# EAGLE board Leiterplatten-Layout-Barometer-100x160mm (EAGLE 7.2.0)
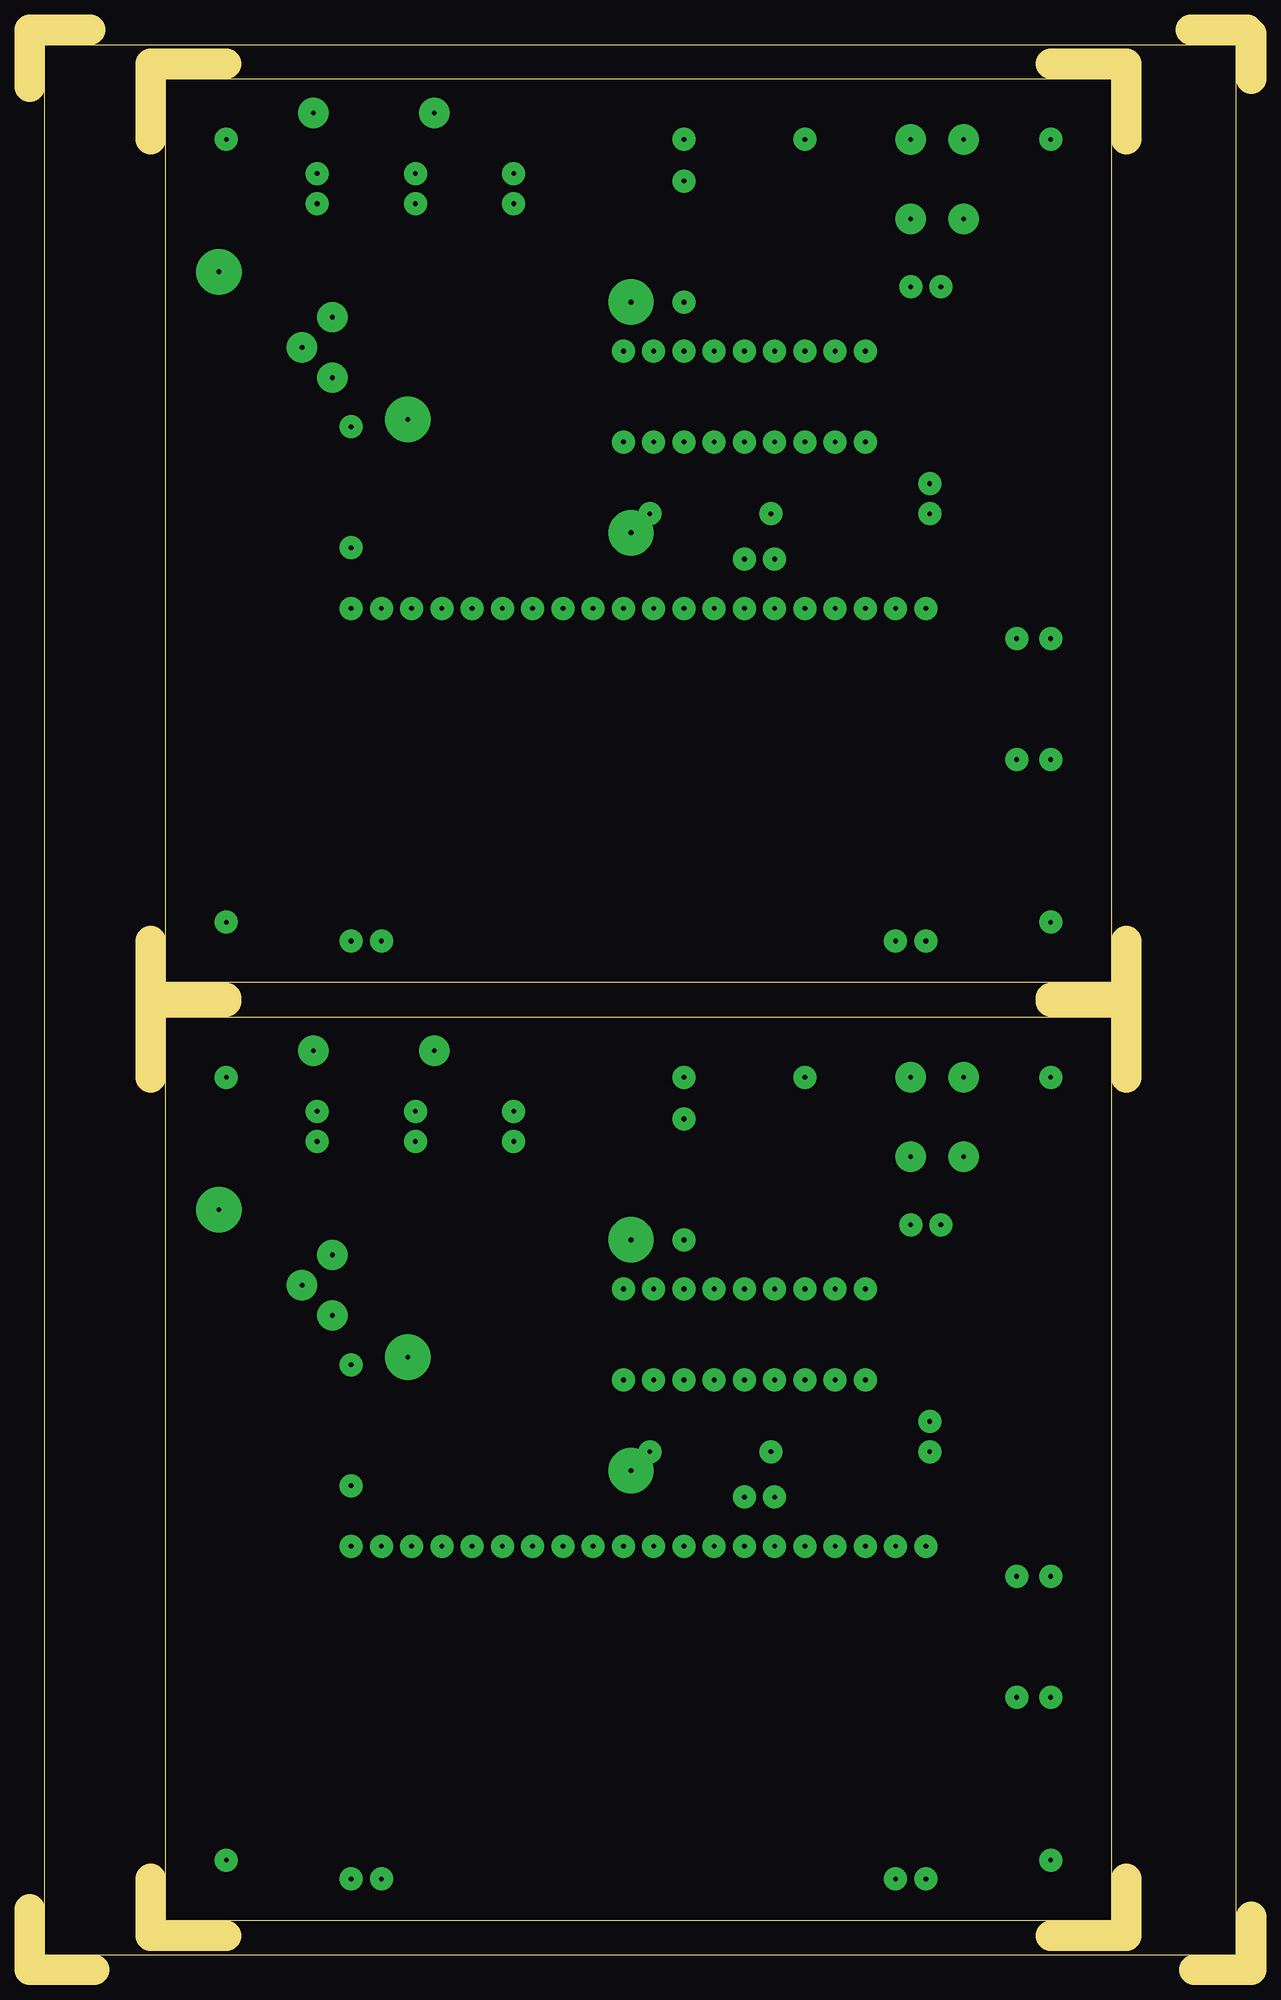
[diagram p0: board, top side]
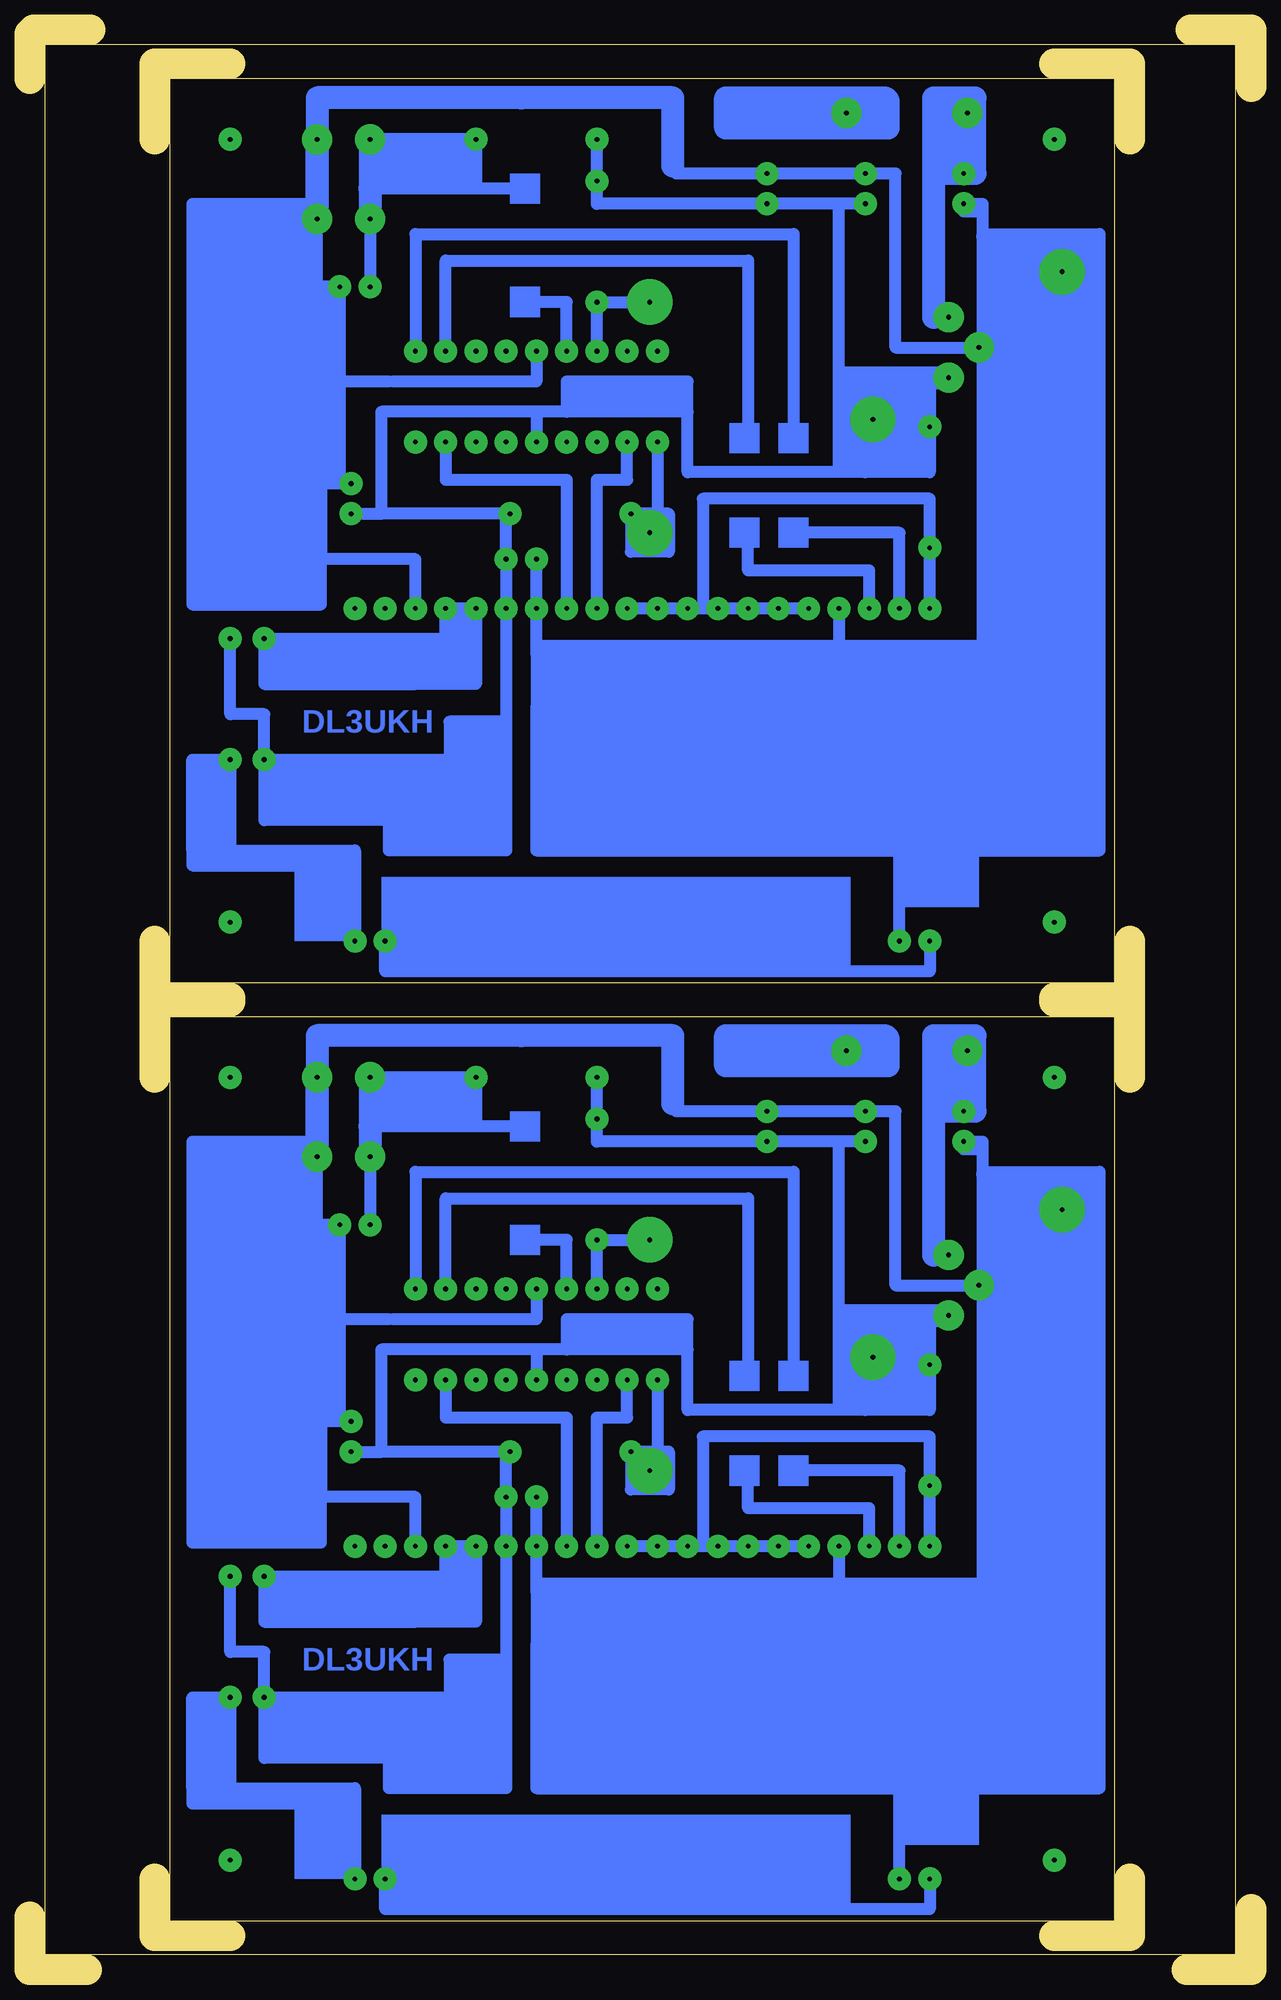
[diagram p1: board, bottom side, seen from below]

Size 102.55 x 162.88 mm. Coordinates in mm from the lower left corner, seen from the top.
Outline: 5.4,0 0.32,0
Outline: 0,0 0,5.08
Outline: 97.79,0 102.55,0 102.55,4.45
Outline: 5.08,162.88 0,162.88 0,158.12
Outline: 102.55,158.75 102.55,162.56
Outline: 97.47,162.88 102.23,162.88
Outline: 92.08,153.67 92.08,160.02 85.72,160.02
Outline: 92.08,86.36 92.08,81.6 85.72,81.6
Outline: 16.51,81.6 10.16,81.6 10.16,86.36
Outline: 10.16,153.67 10.16,160.02 16.51,160.02
Outline: 92.08,74.93 92.08,81.28 85.72,81.28
Outline: 92.08,7.62 92.08,2.86 85.72,2.86
Outline: 16.51,2.86 10.16,2.86 10.16,7.62
Outline: 10.16,74.93 10.16,81.28 16.51,81.28
Outline: 1.27,1.27 101.28,1.27 101.28,161.61 1.27,161.61 1.27,1.27
Outline: 90.8,158.75 90.8,82.87 11.43,82.87 11.43,158.75 90.8,158.75
Outline: 90.8,80.01 90.8,4.13 11.43,4.13 11.43,80.01 90.8,80.01
Copper layers (1*16): Top 0.035mm / dielectric 1.5mm / Bottom 0.035mm
Design rules "default": minimum track width 10mil, minimum drill 24mil, track to track 8mil, track to pad 8mil, pad to pad 8mil, via to via 8mil, smd to smd 8mil, copper to edge 40mil, drill to drill 8mil, minimum pad ring 10mil, minimum via ring 8mil, stop-mask expansion 4mil, vias tented up to drill 0mil, thermal gap 10mil

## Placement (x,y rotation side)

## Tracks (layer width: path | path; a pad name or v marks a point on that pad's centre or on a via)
S$1  (via drill 0.4 pad 1.93)
  Bottom 1.016: v26.99,7.62 26.99,5.08 72.71,5.08 v72.71,7.62
S$2  (via drill 0.4 pad 1.93)
  other vias: 42.23,114.3
S$3  (via drill 0.4 pad 1.93)
  Bottom 1.016: v26.99,86.36 26.99,83.82 72.71,83.82 v72.71,86.36
S$4  (via drill 0.4 pad 1.93, 0.4 pad 2.54)
  Bottom 1.016: 21.91,136.21 v22.86,136.21 29.84,136.21 29.84,150.81 v32.38,150.81 48.26,150.81 | 21.91,136.21 21.91,108.9 23.5,96.52 | v29.53,86.36 29.53,96.52 | 29.53,96.52 60.01,96.52 | 60.01,96.52 60.01,106.05 | 60.01,110.49 60.01,111.12 | 60.01,111.12 v60.01,114.3 v60.01,118.43 | 60.01,96.52 60.01,93.98 23.81,93.98 | 23.5,96.52 29.53,96.52 | 23.5,96.52 23.5,93.98 12.7,93.98 12.7,145.73 22.54,145.73 | 51.75,110.49 50.8,110.49 50.8,106.05 60.01,106.05 | 51.75,110.49 60.01,110.49 | 60.01,110.49 60.01,106.05 | 51.75,109.22 51.75,110.49 | v15.88,142.56 22.54,145.73 | 21.91,136.21 22.54,145.73 | 22.22,111.12 60.01,111.12
S$5
  Bottom 1.016: 34.61,114.3 34.61,95.57
S$6  (via drill 0.4 pad 1.93, 0.4 pad 3.81)
  Bottom 1.016: v54.93,135.89 v54.93,140.02 v50.48,140.02
S$7  (via drill 0.4 pad 1.93)
  other vias: 42.23,35.56
S$8  (via drill 0.4 pad 1.93)
  other vias: 16.51,87.95
S$9  (via drill 0.4 pad 1.93)
  other vias: 16.51,153.67
S$10
  Bottom 1.016: 75.56,156.84 75.56,157.48 | 75.56,157.48 78.74,157.48 | 61.28,157.16 58.42,157.48 | 58.42,157.48 75.56,157.48 | 58.42,157.48 48.58,157.48 48.58,157.16
  Bottom 1.93: 61.28,157.16 78.1,157.16 | 48.58,151.45 48.58,157.16 78.42,157.16 78.42,147
S$11  (via drill 0.4 pad 1.93)
  other vias: 44.77,114.3
S$12  (via drill 0.4 pad 1.93)
  other vias: 57.47,128.27
S$13  (via drill 0.4 pad 1.93)
  other vias: 44.77,35.56
S$14  (via drill 0.4 pad 1.93)
  Bottom 1.016: v54.93,114.3 54.93,125.09 52.39,125.09 v52.39,128.27
S$15  (via drill 0.4 pad 1.93)
  other vias: 34.61,114.3
S$16  (via drill 0.4 pad 1.93, 0.4 pad 2.54)
  Bottom 1.016: v73.98,153.67 v65.09,153.67 65.09,149.54 | 60.96,149.54 65.09,149.54 | 65.09,149.54 73.98,149.54 | v73.98,147 v73.98,141.29
  Bottom 1.93: v73.98,153.67 73.98,149.54 v73.98,147
S$17  (via drill 0.4 pad 1.93)
  Bottom 1.016: v60.01,135.89 60.01,133.35 72.07,133.35
S$18  (via drill 0.4 pad 1.93)
  other vias: 54.93,128.27
S$19  (via drill 0.4 pad 1.93, 0.4 pad 3.81)
  Bottom 1.016: v49.85,128.27 49.85,122.24 v52.07,122.24 | 48.9,122.24 v50.48,120.65 52.07,119.06 | 48.9,122.24 v52.07,122.24 | v52.07,122.24 52.07,119.06 | 48.9,122.24 48.9,119.06 52.07,119.06
  other vias: 52.39,135.89
S$20  (via drill 0.4 pad 1.93)
  other vias: 65.09,128.27
S$21  (via drill 0.4 pad 1.93)
  Bottom 1.016: v29.53,35.56 29.53,41.91 38.42,41.91
S$22  (via drill 0.4 pad 1.93, 0.4 pad 2.54)
  Bottom 1.016: v78.42,147 78.42,141.29 v76.52,141.29 76.52,125.09
  Bottom 1.93: 81.28,147 v78.42,147 v78.42,153.67
S$23  (via drill 0.4 pad 3.81)
  other vias: 15.88,142.56
S$24  (via drill 0.4 pad 1.93)
  Bottom 1.016: v67.63,128.27 67.63,125.09 57.47,125.09 v57.47,114.3
S$25  (via drill 0.4 pad 1.93)
  other vias: 72.71,114.3
S$26  (via drill 0.4 pad 1.93)
  other vias: 75.25,114.3
S$27  (via drill 0.4 pad 3.81)
  other vias: 31.75,130.18
S$28  (via drill 0.4 pad 1.93)
  Bottom 1.016: v67.63,135.89 67.63,143.51 42.23,143.51 42.23,128.27
S$29  (via drill 0.4 pad 1.93)
  other vias: 85.72,87.95
S$30  (via drill 0.4 pad 1.93)
  Bottom 1.016: 70.17,107.95 82.87,107.95 v82.87,111.76 70.17,111.76 | 65.09,111.76 v65.09,114.3 v67.63,114.3 67.63,110.49 | 65.09,111.76 65.09,110.49 | 65.09,110.49 67.63,110.49 | 67.63,110.49 70.17,110.49 | 70.17,110.49 70.17,111.76 | 70.17,107.95 70.17,110.49 | 65.09,110.49 65.09,107.95 70.17,107.95 | 70.17,111.76 65.09,111.76
S$31  (via drill 0.4 pad 1.93)
  Bottom 1.016: v26.99,35.56 v26.99,40.64 26.99,44.77 46.04,44.77 46.04,35.56 | 85.72,15.24 75.25,15.24 v75.25,7.62 | 85.72,15.24 v85.72,22.86 88.9,22.86 88.9,15.24 | 85.72,15.24 88.9,15.24 | 88.9,15.24 88.9,13.97 79.38,13.97 | v52.39,35.56 v47.31,35.56 46.04,35.56 | 46.04,35.56 v39.69,35.56 v37.15,35.56
S$32  (via drill 0.4 pad 1.93)
  Bottom 1.016: v57.47,135.89 57.47,140.02 60.96,140.02
S$33  (via drill 0.4 pad 1.93)
  Bottom 1.016: 38.42,128.27 38.42,145.73 70.17,145.73 v70.17,135.89
S$34  (via drill 0.4 pad 1.93)
  other vias: 85.72,153.67
S$35  (via drill 0.4 pad 1.93)
  other vias: 49.85,135.89 70.17,128.27
S$36  (via drill 0.4 pad 1.93)
  other vias: 49.85,35.56
S$37
  Bottom 1.016: 78.74,148.27 88.9,148.27 88.9,114.62 78.1,114.62 78.1,118.11
S$38  (via drill 0.4 pad 1.93)
  Bottom 1.016: v29.53,114.3 29.53,120.65 38.42,120.65
S$39  (via drill 0.4 pad 1.93)
  Bottom 1.016: v85.72,111.76 85.72,105.41 82.87,105.41 v82.87,101.6 | 67.31,100.96 67.31,104.77 62.55,104.77 | v82.87,101.6 62.87,101.6 | v82.87,101.6 82.87,96.52 62.55,96.52 | 62.55,104.77 v62.55,114.3 v62.55,118.43 62.55,122.24 | 72.39,96.84 72.39,93.98 62.55,93.98 62.55,96.52 | 62.55,104.77 62.55,96.52 | 59.69,130.81 73.02,130.81 73.02,122.24 | 62.55,122.24 73.02,122.24 | v62.23,122.24 62.55,122.24 | v75.56,122.24 73.02,122.24
S$40  (via drill 0.4 pad 1.93)
  other vias: 40.64,150.81
S$41  (via drill 0.4 pad 1.93)
  other vias: 62.55,135.89
S$42  (via drill 0.4 pad 1.93)
  Bottom 1.016: 76.83,135.89 78.1,135.89 | 78.1,135.89 87.63,135.89 | 87.63,135.89 88.9,135.89 | 87.63,135.89 87.63,118.43 | v70.17,114.3 70.17,118.43 78.1,118.43 | 78.1,118.43 88.58,118.43 | 78.1,135.89 78.1,118.43
S$43
  Bottom 1.016: 72.39,133.35 78.74,133.35
S$44  (via drill 0.4 pad 1.93)
  Bottom 1.016: 42.23,120.65 42.23,117.47 32.07,117.47 v32.07,114.3
S$45  (via drill 0.4 pad 1.93)
  other vias: 65.09,135.89
S$46  (via drill 0.4 pad 1.93)
  Bottom 1.016: v75.56,124.78 78.74,124.78
S$47  (via drill 0.4 pad 1.93)
  Bottom 1.016: v26.99,114.3 v26.99,119.38 26.99,123.51 46.04,123.51 46.04,114.3 | 85.72,93.98 75.25,93.98 v75.25,86.36 | 85.72,93.98 v85.72,101.6 88.9,101.6 88.9,93.98 | 85.72,93.98 88.9,93.98 | 88.9,93.98 88.9,92.71 79.38,92.71 | v52.39,114.3 v47.31,114.3 46.04,114.3 | 46.04,114.3 v39.69,114.3 v37.15,114.3
S$48  (via drill 0.4 pad 1.93)
  other vias: 49.85,114.3
S$49  (via drill 0.4 pad 1.93, 0.4 pad 2.54)
  Bottom 1.93: 23.5,157.16 23.5,150.81 v24.13,150.81 25.08,150.81 | 25.08,157.16 25.08,154.94 | 25.08,154.94 v23.81,155.89 | 25.08,157.16 26.67,157.16 26.67,150.81 25.08,150.81 | 25.08,157.16 23.18,157.16 23.18,150.81 | 25.08,154.94 25.08,150.81 | 25.08,150.81 25.4,157.16
S$50
  Bottom 1.93: 30.48,154.62 44.13,154.62 44.13,157.16
S$51  (via drill 0.4 pad 1.93, 0.4 pad 2.54)
  Bottom 2.54: v33.97,155.89 31.11,156.84 34.29,156.84 | 34.29,156.84 v33.97,155.89 | v33.97,155.89 30.8,154.94 30.8,156.84 v33.97,155.89 | v33.97,155.89 40.01,154.94 43.82,156.84 34.29,156.84
  other vias: 15.88,142.56 15.88,142.56
S$52  (via drill 0.4 pad 1.93, 0.4 pad 2.54)
  Bottom 1.016: v26.99,129.54 26.99,125.73 32.38,125.73 | 32.38,125.73 47.31,125.73 47.31,130.81 | 47.31,130.81 57.47,130.81 | 57.47,130.81 60.01,130.81 v60.01,128.27 | v25.4,133.67 26.99,133.35 | 26.99,133.35 v26.99,129.54 | v26.99,129.54 32.38,129.54 | 32.38,129.54 32.38,125.73 | 26.99,133.35 32.38,133.35 | 32.38,133.35 32.38,129.54 | 32.38,133.35 34.61,126.05 34.61,148.27 | 47.31,130.81 47.31,133.35 57.47,133.35 57.47,130.81
  Bottom 1.93: 33.97,133.67 v25.4,133.67
S$53  (via drill 0.4 pad 2.54)
  Bottom 1.93: v25.4,138.75 26.67,138.75 26.67,150.5
S$54  (via drill 0.4 pad 1.93)
  Bottom 1.016: v32.38,148.27 v40.64,148.27 54.93,148.27 v54.93,150.18 v54.93,153.67
S$55
  Bottom 1.93: 21.91,145.1 21.91,144.46
S$56  (via drill 0.4 pad 1.93)
  Bottom 1.016: 22.54,147.64 22.54,109.85 | v24.13,148.27 22.54,148.27 22.54,147.64 | 24.13,147.64 22.54,147.64
S$57  (via drill 0.4 pad 1.93)
  other vias: 62.55,128.27
S$58  (via drill 0.4 pad 1.93)
  Bottom 1.016: v54.93,35.56 54.93,46.36 52.39,46.36 v52.39,49.53
S$59  (via drill 0.4 pad 1.93)
  other vias: 54.93,49.53
S$60  (via drill 0.4 pad 1.93)
  other vias: 72.71,35.56
S$61  (via drill 0.4 pad 1.93)
  other vias: 75.25,35.56
S$62  (via drill 0.4 pad 1.93)
  Bottom 1.016: 70.17,29.21 82.87,29.21 v82.87,33.02 70.17,33.02 | 65.09,33.02 v65.09,35.56 v67.63,35.56 67.63,31.75 | 65.09,33.02 65.09,31.75 | 65.09,31.75 67.63,31.75 | 67.63,31.75 70.17,31.75 | 70.17,31.75 70.17,33.02 | 70.17,29.21 70.17,31.75 | 65.09,31.75 65.09,29.21 70.17,29.21 | 70.17,33.02 65.09,33.02
S$63  (via drill 0.4 pad 1.93)
  other vias: 57.47,49.53
S$64  (via drill 0.4 pad 1.93)
  other vias: 62.55,49.53
S$65  (via drill 0.4 pad 1.93)
  other vias: 65.09,49.53
S$66  (via drill 0.4 pad 1.93)
  Bottom 1.016: v67.63,49.53 67.63,46.36 57.47,46.36 v57.47,35.56
S$67  (via drill 0.4 pad 1.93)
  other vias: 62.55,57.15
S$68  (via drill 0.4 pad 1.93)
  Bottom 1.016: v57.47,57.15 57.47,61.28 60.96,61.28
S$69  (via drill 0.4 pad 1.93, 0.4 pad 3.81)
  Bottom 1.016: v54.93,57.15 v54.93,61.28 v50.48,61.28
S$70  (via drill 0.4 pad 1.93)
  Bottom 1.016: 38.42,49.53 38.42,66.99 70.17,66.99 v70.17,57.15
S$71  (via drill 0.4 pad 1.93)
  other vias: 49.85,57.15 70.17,49.53
S$72  (via drill 0.4 pad 1.93, 0.4 pad 3.81)
  Bottom 1.016: v49.85,49.53 49.85,43.5 v52.07,43.5 | 48.9,43.5 v50.48,41.91 52.07,40.32 | 48.9,43.5 v52.07,43.5 | v52.07,43.5 52.07,40.32 | 48.9,43.5 48.9,40.32 52.07,40.32
  other vias: 52.39,57.15
S$73  (via drill 0.4 pad 3.81)
  other vias: 31.75,51.44
S$74  (via drill 0.4 pad 1.93)
  other vias: 85.72,9.21
S$75  (via drill 0.4 pad 1.93)
  other vias: 85.72,74.93
S$76
  Bottom 1.016: 75.56,78.1 75.56,78.74 | 75.56,78.74 78.74,78.74 | 61.28,78.42 58.42,78.74 | 58.42,78.74 75.56,78.74 | 58.42,78.74 48.58,78.74 48.58,78.42
  Bottom 1.93: 61.28,78.42 78.1,78.42 | 48.58,72.71 48.58,78.42 78.42,78.42 78.42,68.26
S$77
  Bottom 1.016: 78.74,69.53 88.9,69.53 88.9,35.88 78.1,35.88 78.1,39.37
S$78  (via drill 0.4 pad 1.93)
  Bottom 1.016: v60.01,57.15 60.01,54.61 72.07,54.61
S$79  (via drill 0.4 pad 1.93)
  Bottom 1.016: 42.23,41.91 42.23,38.74 32.07,38.74 v32.07,35.56
S$80  (via drill 0.4 pad 1.93)
  other vias: 34.61,35.56
S$81  (via drill 0.4 pad 1.93, 0.4 pad 2.54)
  Bottom 1.016: 21.91,57.47 v22.86,57.47 29.84,57.47 29.84,72.07 v32.38,72.07 48.26,72.07 | 21.91,57.47 21.91,30.16 23.5,17.78 | v29.53,7.62 29.53,17.78 | 29.53,17.78 60.01,17.78 | 60.01,17.78 60.01,27.3 | 60.01,31.75 60.01,32.38 | 60.01,32.38 v60.01,35.56 v60.01,39.69 | 60.01,17.78 60.01,15.24 23.81,15.24 | 23.5,17.78 29.53,17.78 | 23.5,17.78 23.5,15.24 12.7,15.24 12.7,66.99 22.54,66.99 | 51.75,31.75 50.8,31.75 50.8,27.3 60.01,27.3 | 51.75,31.75 60.01,31.75 | 60.01,31.75 60.01,27.3 | 51.75,30.48 51.75,31.75 | v15.88,63.82 22.54,66.99 | 21.91,57.47 22.54,66.99 | 22.22,32.38 60.01,32.38
S$82  (via drill 0.4 pad 1.93)
  Bottom 1.016: v67.63,57.15 67.63,64.77 42.23,64.77 42.23,49.53
S$83  (via drill 0.4 pad 1.93)
  other vias: 65.09,57.15
S$84  (via drill 0.4 pad 1.93)
  other vias: 16.51,9.21
S$85  (via drill 0.4 pad 1.93)
  other vias: 16.51,74.93
S$86  (via drill 0.4 pad 3.81)
  other vias: 15.88,63.82
S$87  (via drill 0.4 pad 1.93)
  other vias: 40.64,72.07
S$88  (via drill 0.4 pad 2.54)
  Bottom 1.93: v25.4,60.01 26.67,60.01 26.67,71.75
S$89  (via drill 0.4 pad 1.93, 0.4 pad 2.54)
  Bottom 1.93: 23.5,78.42 23.5,72.07 v24.13,72.07 25.08,72.07 | 25.08,78.42 25.08,76.2 | 25.08,76.2 v23.81,77.15 | 25.08,78.42 26.67,78.42 26.67,72.07 25.08,72.07 | 25.08,78.42 23.18,78.42 23.18,72.07 | 25.08,76.2 25.08,72.07 | 25.08,72.07 25.4,78.42
S$90
  Bottom 1.93: 30.48,75.88 44.13,75.88 44.13,78.42
S$91  (via drill 0.4 pad 1.93, 0.4 pad 2.54)
  Bottom 2.54: v33.97,77.15 31.11,78.1 34.29,78.1 | 34.29,78.1 v33.97,77.15 | v33.97,77.15 30.8,76.2 30.8,78.1 v33.97,77.15 | v33.97,77.15 40.01,76.2 43.82,78.1 34.29,78.1
  other vias: 15.88,63.82 15.88,63.82
S$92  (via drill 0.4 pad 1.93, 0.4 pad 2.54)
  Bottom 1.016: v26.99,50.8 26.99,46.99 32.38,46.99 | 32.38,46.99 47.31,46.99 47.31,52.07 | 47.31,52.07 57.47,52.07 | 57.47,52.07 60.01,52.07 v60.01,49.53 | v25.4,54.93 26.99,54.61 | 26.99,54.61 v26.99,50.8 | v26.99,50.8 32.38,50.8 | 32.38,50.8 32.38,46.99 | 26.99,54.61 32.38,54.61 | 32.38,54.61 32.38,50.8 | 32.38,54.61 34.61,47.31 34.61,69.53 | 47.31,52.07 47.31,54.61 57.47,54.61 57.47,52.07
  Bottom 1.93: 33.97,54.93 v25.4,54.93
S$93  (via drill 0.4 pad 1.93)
  Bottom 1.016: v32.38,69.53 v40.64,69.53 54.93,69.53 v54.93,71.44 v54.93,74.93
S$94  (via drill 0.4 pad 1.93)
  Bottom 1.016: 22.54,68.9 22.54,31.11 | v24.13,69.53 22.54,69.53 22.54,68.9 | 24.13,68.9 22.54,68.9
S$95
  Bottom 1.93: 21.91,66.36 21.91,65.72
S$96
  Bottom 1.016: 34.61,35.56 34.61,16.83
S$97  (via drill 0.4 pad 1.93, 0.4 pad 2.54)
  Bottom 1.016: v73.98,74.93 v65.09,74.93 65.09,70.8 | 60.96,70.8 65.09,70.8 | 65.09,70.8 73.98,70.8 | v73.98,68.26 v73.98,62.55
  Bottom 1.93: v73.98,74.93 73.98,70.8 v73.98,68.26
S$98
  Bottom 1.016: 72.39,54.61 78.74,54.61
S$99  (via drill 0.4 pad 1.93)
  Bottom 1.016: v85.72,33.02 85.72,26.67 82.87,26.67 v82.87,22.86 | 67.31,22.22 67.31,26.04 62.55,26.04 | v82.87,22.86 62.87,22.86 | v82.87,22.86 82.87,17.78 62.55,17.78 | 62.55,26.04 v62.55,35.56 v62.55,39.69 62.55,43.5 | 72.39,18.1 72.39,15.24 62.55,15.24 62.55,17.78 | 62.55,26.04 62.55,17.78 | 59.69,52.07 73.02,52.07 73.02,43.5 | 62.55,43.5 73.02,43.5 | v62.23,43.5 62.55,43.5 | v75.56,43.5 73.02,43.5
S$100  (via drill 0.4 pad 1.93)
  Bottom 1.016: v75.56,46.04 78.74,46.04
S$101  (via drill 0.4 pad 1.93)
  Bottom 1.016: 76.83,57.15 78.1,57.15 | 78.1,57.15 87.63,57.15 | 87.63,57.15 88.9,57.15 | 87.63,57.15 87.63,39.69 | v70.17,35.56 70.17,39.69 78.1,39.69 | 78.1,39.69 88.58,39.69 | 78.1,57.15 78.1,39.69
S$102  (via drill 0.4 pad 1.93, 0.4 pad 2.54)
  Bottom 1.016: v78.42,68.26 78.42,62.55 v76.52,62.55 76.52,46.36
  Bottom 1.93: 81.28,68.26 v78.42,68.26 v78.42,74.93
(copper drawn outside any net)
  shapes: Bottom area x70

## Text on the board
Bottom: DL3UKH | DL3UKH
